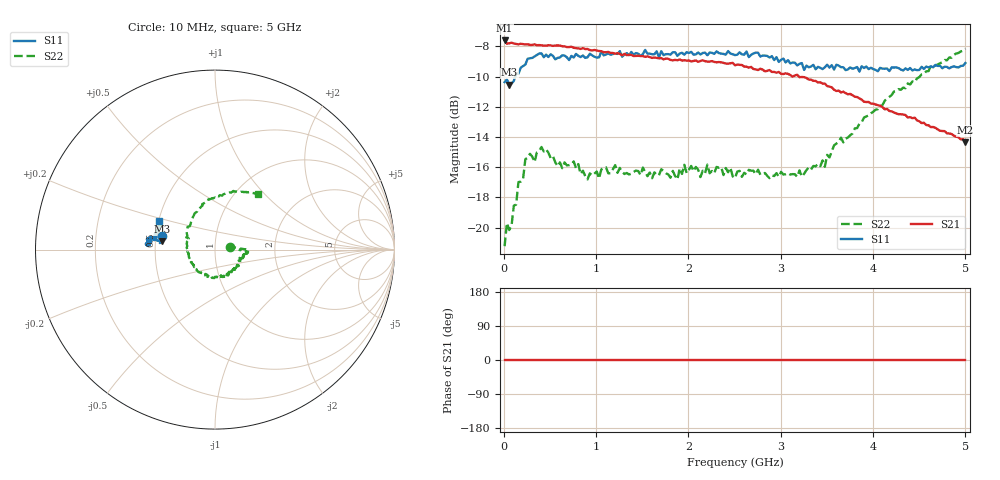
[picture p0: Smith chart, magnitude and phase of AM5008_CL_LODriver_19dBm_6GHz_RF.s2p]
!Keysight Technologies,N5245B,MY58422270,A.16.20.02
!Mixer S2P File: Scalar Mixer Measurement
!Calibration State: On
!Parameters: Stimulus Freq, S11, SC21, SC12, S22
# Hz  S  DB  R  50.0
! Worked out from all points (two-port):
!   201 points, 10 MHz to 5 GHz, reference 50 ohm
!   highest |S21| = -7.61 dB at 10 MHz (marker M1); lowest = -14.4 dB at 5 GHz (marker M2)
!   |S21| within 3 dB of the highest: start of sweep to 3.5 GHz
!   lowest |S11| = -10.5 dB at 59.9 MHz (marker M3), VSWR 1.85, Z = 27.2 + j2.8 ohm
!   |S11| at or under -10 dB: start of sweep to 124.6 MHz
!   |S22| runs from -21.2 to -8.2 dB; largest |S21 - S12| = 0.42
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1e7  -10.37 165.8  -7.61 0.0  -200.00 90.0  -21.23 8.8
3.495e7  -10.19 173.3  -7.83 0.0  -200.00 90.0  -19.69 2.9
5.99e7  -10.54 170.9  -7.80 0.0  -200.00 90.0  -20.16 4.5
1.3475e8  -9.80 171.2  -7.84 0.0  -200.00 90.0  -18.47 2.2
1.597e8  -9.82 171.1  -7.87 0.0  -200.00 90.0  -16.99 -1.5
2.8445e8  -8.79 171.5  -7.90 0.0  -200.00 90.0  -15.11 -1.4
3.3435e8  -8.67 170.9  -7.87 0.0  -200.00 90.0  -15.66 -0.9
4.092e8  -8.46 172.1  -7.94 0.0  -200.00 90.0  -14.66 -3.8
5.8385e8  -8.76 173.5  -7.94 0.0  -200.00 90.0  -15.94 -10.3
8.583e8  -8.60 175.4  -8.12 0.0  -200.00 90.0  -16.23 -17.3
1.68165e9  -8.72 174.4  -8.79 0.0  -200.00 90.0  -16.54 -50.2
1.88125e9  -8.63 174.4  -8.92 0.0  -200.00 90.0  -16.81 -59.9
1.9561e9  -8.55 174.5  -8.92 0.0  -200.00 90.0  -15.84 -62.8
2.13075e9  -8.53 172.9  -8.97 0.0  -200.00 90.0  -16.66 -76.6
2.2056e9  -8.59 172.7  -9.01 0.0  -200.00 90.0  -15.83 -82.0
2.505e9  -8.58 172.3  -9.25 0.0  -200.00 90.0  -16.73 -111.5
3.3533e9  -9.22 167.3  -10.28 0.0  -200.00 90.0  -15.92 169.3
3.47805e9  -9.39 167.0  -10.47 0.0  -200.00 90.0  -15.97 157.1
3.6527e9  -9.38 164.8  -11.05 0.0  -200.00 90.0  -14.04 140.0
4.17665e9  -9.63 159.4  -12.28 0.0  -200.00 90.0  -11.35 100.2
4.62575e9  -9.32 155.1  -13.35 0.0  -200.00 90.0  -9.31 72.6
5e9  -9.10 153.5  -14.36 0.0  -200.00 90.0  -8.15 52.7
